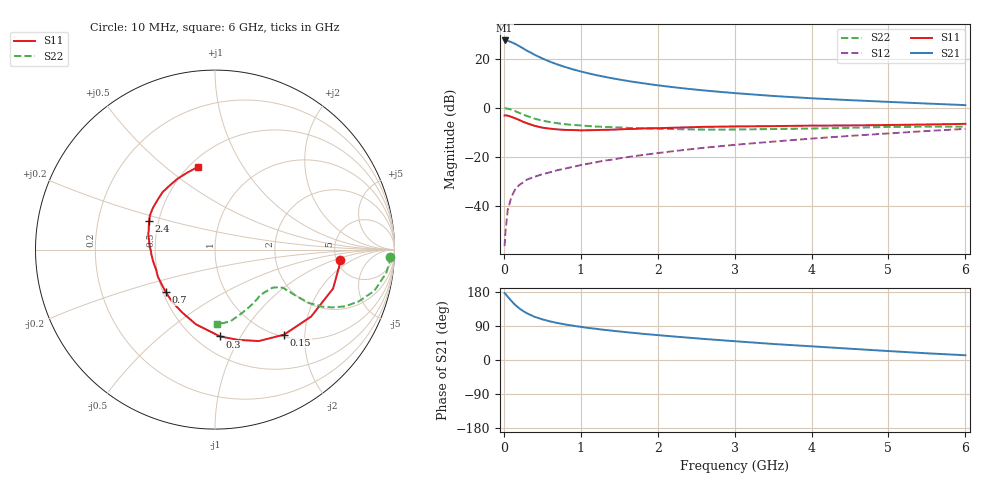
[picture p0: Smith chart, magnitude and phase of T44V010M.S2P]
! Infineon Technologies  Discrete & RF Semiconductors
! BFR182T
! Si NPN RF Bipolar Junction Transistor in SC75
! VCE = 4 V  IC = 10 mA
! Common Emitter S-Parameters:  October  1999
# GHz  S  MA  R  50
!  f  S11  S21  S12  S22
! GHz  MAG  ANG  MAG  ANG  MAG  ANG  MAG  ANG
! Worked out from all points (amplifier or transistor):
!   36 points, 10 MHz to 6 GHz, reference 50 ohm
!   highest |S21| = 27.5 dB at 10 MHz (marker M1)
!   |S21| within 3 dB of that: start of sweep to 237.3 MHz
!   unconditionally stable (mu >= 1): 1.023 GHz to 3.811 GHz
!   at 250 MHz: K = 0.45, MSG = 27.4 dB, |S12| = -30.4 dB
!   at 1.4 GHz: K = 1.07, MAG = 15.1 dB, |S12| = -21.2 dB
!   at 6 GHz: K = 0.85, MSG = 4.8 dB, |S12| = -8.6 dB
!   lowest NFmin = 1.50 dB at 450 MHz
!   S11 on the Smith chart (normalised r, x): 10 MHz: 5.32, -1.18; 150 MHz: 1.04, -1.57; 300 MHz: 0.65, -0.82; 700 MHz: 0.52, -0.28; 2.4 GHz: 0.44, +0.17; 6 GHz: 0.55, +0.66
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0.01  0.6963 -4.7  23.74 176.4  0.0015 84.4  0.9734 -2.3
0.02  0.7015 -5.9  23.57 174.9  0.0028 88.8  0.9788 -3.0
0.05  0.6929 -18.2  23.32 167.0  0.0082 80.9  0.9633 -7.7
0.1  0.6527 -34.9  21.89 155.5  0.0154 76.3  0.9173 -14.5
0.15  0.6104 -50.9  20.1 144.9  0.0219 68.8  0.8514 -19.8
0.2  0.565 -64.4  18.2 136.4  0.0266 66.3  0.7905 -23.6
0.25  0.519 -75.7  16.36 129.3  0.0301 61.2  0.7291 -26.2
0.3  0.4849 -86.6  14.72 123.3  0.0343 60.5  0.6807 -27.9
0.4  0.4296 -104.4  12.13 114.0  0.0392 58.3  0.6007 -29.6
0.5  0.3943 -118.1  10.2 107.3  0.0442 58.5  0.5491 -29.7
0.6  0.3758 -129.6  8.741 101.9  0.0482 59.4  0.5113 -29.7
0.7  0.3627 -139.2  7.654 97.5  0.0534 60.5  0.4838 -29.5
0.9  0.3523 -154.8  6.087 90.5  0.0625 62.2  0.4465 -29.4
1.1  0.3489 -166.6  5.062 84.6  0.0726 63.6  0.4258 -29.8
1.3  0.3553 -175.7  4.335 79.7  0.0835 64.4  0.4083 -30.7
1.6  0.3692 173.7  3.556 73.2  0.0982 65.6  0.3909 -32.7
2.2  0.3929 159.8  2.642 62.2  0.1302 66.4  0.3692 -38.8
2.4  0.4007 156.2  2.437 58.9  0.1414 66.2  0.3631 -41.3
3.5  0.4235 138.8  1.747 42.3  0.2043 63.6  0.369 -55.9
4.5  0.4368 125.8  1.435 29.8  0.2674 59.2  0.391 -70.5
5.5  0.4564 109.4  1.224 17.7  0.3364 53.8  0.4123 -83.3
6  0.471 101.4  1.136 12.5  0.3722 50.2  0.4124 -88.4
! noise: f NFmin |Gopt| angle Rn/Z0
0.45  1.5  0.26  43  0.28
0.9  1.6  0.24  87  0.22
1.8  2.1  0.2  170  0.2
